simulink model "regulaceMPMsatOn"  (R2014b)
settings: Solver=ode45  StartTime=0.0  StopTime=50  RelTol=1e-3
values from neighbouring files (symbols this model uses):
  par = [0.2728 0.1079 0.3077 0.0546 0.1370 0.0320 0.1151 0.0357]    [regulaceMPM.m]    (also in SITOrizeniP.m = [-0.0536 0.05 0.13 0.006 -0.0545 0.1 0.16 0.1746 -0.058     ; SITOrizeniPD.m = [-0.0536 0.05 0.13 0.006 -0.0545 0.1 0.16 0.1746 -0.058     ; regulace1DoF.m; regulace2DoF.m)
undefined symbols (not defined in the file or in its folder): D, magnitude, N, P
libraries: simulink x8

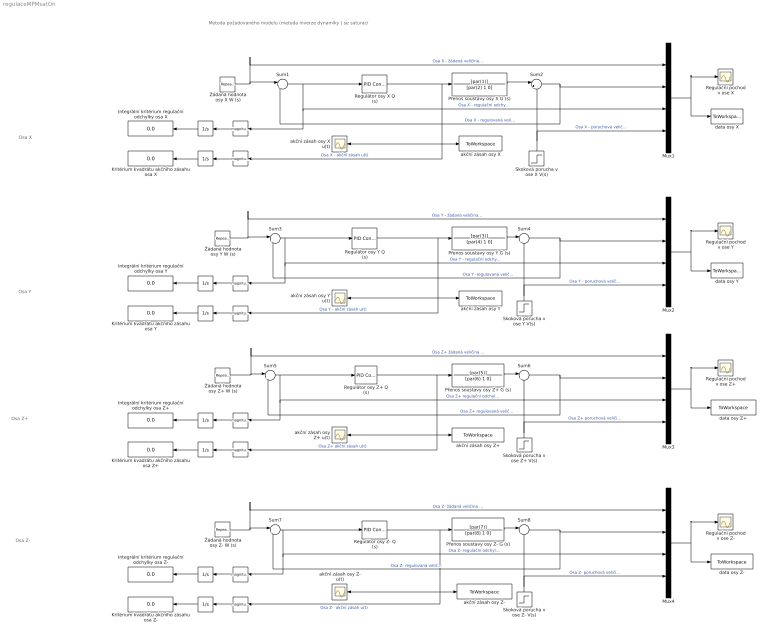
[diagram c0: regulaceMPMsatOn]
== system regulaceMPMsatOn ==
  note: Osa X
  note: Metoda požadovaného modelu (metoda inverze dynamiky ) se saturací
  note: Osa Y
  note: Osa Z+
  note: Osa Z-
  " " : Math  Operator=magnitude^2
  "  " : Integrator
  "   " : Integrator
  "     " : Integrator
  "      " : Math  Operator=magnitude^2
  "       " : Math  Operator=magnitude^2
  "        " : Integrator
  "          " : Integrator
  "           " : Math  Operator=magnitude^2
  "             " : Math  Operator=magnitude^2
  "              " : Integrator
  "                 " : Math  Operator=magnitude^2
  "                            " : Integrator
  "                               " : Math  Operator=magnitude^2
  "                                     " : Math  Operator=magnitude^2
  "                                       " : Integrator
  Integrální kritérium regulační odchylky osa X : Display
  Integrální kritérium regulační odchylky osa Y : Display
  Integrální kritérium regulační odchylky osa Z+ : Display
  Integrální kritérium regulační odchylky osa Z- : Display
  Kritérium kvadrátu akčního zásahu osa X : Display
  Kritérium kvadrátu akčního zásahu osa Y : Display
  Kritérium kvadrátu akčního zásahu osa Z+ : Display
  Kritérium kvadrátu akčního zásahu osa Z- : Display
  Mux{1..4} (4 alike) : Mux
  Přenos soustavy osy X G (s) : TransferFcn  Numerator=[par(1)]  Denominator=[par(2) 1 0]
  Přenos soustavy osy Y G (s) : TransferFcn  Numerator=[par(3)]  Denominator=[par(4) 1 0]
  Přenos soustavy osy Z+ G (s) : TransferFcn  Numerator=[par(5)]  Denominator=[par(6) 1 0]
  Přenos soustavy osy Z- G (s) : TransferFcn  Numerator=[par(7)]  Denominator=[par(8) 1 0]
  Regulační pochod v ose X : Scope
  Regulační pochod v ose Y : Scope
  Regulační pochod v ose Z+ : Scope
  Regulační pochod v ose Z- : Scope
  Regulátor osy X Q (s) : simulink/Continuous/PID Controller  Controller=PID  TimeDomain=Continuous-time  SampleTime=-1  IntegratorMethod=Forward Euler  FilterMethod=Forward Euler  Form=Parallel  P=P(1)  I=0  D=D(1)  N=N(1)  InitialConditionSource=internal  InitialConditionForIntegrator=0  InitialConditionForFilter=0  ExternalReset=none  LimitOutput=on  UpperSaturationLimit=1  LowerSaturationLimit=-1  LinearizeAsGain=on  AntiWindupMode=clamping  Kb=1  TrackingMode=off  Kt=1  PParamMin=[]  PParamMax=[]  IParamMin=[]  IParamMax=[]  DParamMin=[]  DParamMax=[]  NParamMin=[]  NParamMax=[]  KbParamMin=[]  KbParamMax=[]  KtParamMin=[]  KtParamMax=[]  POutMin=[]  POutMax=[]  IOutMin=[]  IOutMax=[]  DOutMin=[]  DOutMax=[]  NOutMin=[]  NOutMax=[]  KbOutMin=[]  KbOutMax=[]  KtOutMin=[]  KtOutMax=[]  IntegratorOutMin=[]  IntegratorOutMax=[]  FilterOutMin=[]  FilterOutMax=[]  SumOutMin=[]  SumOutMax=[]  SumI1OutMin=[]  SumI1OutMax=[]  SumI2OutMin=[]  SumI2OutMax=[]  SumI3OutMin=[]  SumI3OutMax=[]  SumDOutMin=[]  SumDOutMax=[]  SaturationOutMin=[]  SaturationOutMax=[]  IntegratorContinuousStateAttributes=''  IntegratorStateMustResolveToSignalObject=off  IntegratorRTWStateStorageClass=Auto  FilterContinuousStateAttributes=''  FilterStateMustResolveToSignalObject=off  FilterRTWStateStorageClass=Auto  DifferentiatorICPrevScaledInput=0  DifferentiatorOutMin=[]  DifferentiatorOutMax=[]  UseFilter=on
  Regulátor osy Y Q (s) : simulink/Continuous/PID Controller  Controller=PID  TimeDomain=Continuous-time  SampleTime=-1  IntegratorMethod=Forward Euler  FilterMethod=Forward Euler  Form=Parallel  P=P(2)  I=0  D=D(2)  N=N(2)  InitialConditionSource=internal  InitialConditionForIntegrator=0  InitialConditionForFilter=0  ExternalReset=none  LimitOutput=on  UpperSaturationLimit=1  LowerSaturationLimit=-1  LinearizeAsGain=on  AntiWindupMode=clamping  Kb=1  TrackingMode=off  Kt=1  PParamMin=[]  PParamMax=[]  IParamMin=[]  IParamMax=[]  DParamMin=[]  DParamMax=[]  NParamMin=[]  NParamMax=[]  KbParamMin=[]  KbParamMax=[]  KtParamMin=[]  KtParamMax=[]  POutMin=[]  POutMax=[]  IOutMin=[]  IOutMax=[]  DOutMin=[]  DOutMax=[]  NOutMin=[]  NOutMax=[]  KbOutMin=[]  KbOutMax=[]  KtOutMin=[]  KtOutMax=[]  IntegratorOutMin=[]  IntegratorOutMax=[]  FilterOutMin=[]  FilterOutMax=[]  SumOutMin=[]  SumOutMax=[]  SumI1OutMin=[]  SumI1OutMax=[]  SumI2OutMin=[]  SumI2OutMax=[]  SumI3OutMin=[]  SumI3OutMax=[]  SumDOutMin=[]  SumDOutMax=[]  SaturationOutMin=[]  SaturationOutMax=[]  IntegratorContinuousStateAttributes=''  IntegratorStateMustResolveToSignalObject=off  IntegratorRTWStateStorageClass=Auto  FilterContinuousStateAttributes=''  FilterStateMustResolveToSignalObject=off  FilterRTWStateStorageClass=Auto  DifferentiatorICPrevScaledInput=0  DifferentiatorOutMin=[]  DifferentiatorOutMax=[]  UseFilter=on
  Regulátor osy Z+ Q (s) : simulink/Continuous/PID Controller  Controller=PID  TimeDomain=Continuous-time  SampleTime=-1  IntegratorMethod=Forward Euler  FilterMethod=Forward Euler  Form=Parallel  P=P(3)  I=0  D=D(3)  N=N(3)  InitialConditionSource=internal  InitialConditionForIntegrator=0  InitialConditionForFilter=0  ExternalReset=none  LimitOutput=on  UpperSaturationLimit=1  LowerSaturationLimit=-1  LinearizeAsGain=on  AntiWindupMode=clamping  Kb=1  TrackingMode=off  Kt=1  PParamMin=[]  PParamMax=[]  IParamMin=[]  IParamMax=[]  DParamMin=[]  DParamMax=[]  NParamMin=[]  NParamMax=[]  KbParamMin=[]  KbParamMax=[]  KtParamMin=[]  KtParamMax=[]  POutMin=[]  POutMax=[]  IOutMin=[]  IOutMax=[]  DOutMin=[]  DOutMax=[]  NOutMin=[]  NOutMax=[]  KbOutMin=[]  KbOutMax=[]  KtOutMin=[]  KtOutMax=[]  IntegratorOutMin=[]  IntegratorOutMax=[]  FilterOutMin=[]  FilterOutMax=[]  SumOutMin=[]  SumOutMax=[]  SumI1OutMin=[]  SumI1OutMax=[]  SumI2OutMin=[]  SumI2OutMax=[]  SumI3OutMin=[]  SumI3OutMax=[]  SumDOutMin=[]  SumDOutMax=[]  SaturationOutMin=[]  SaturationOutMax=[]  IntegratorContinuousStateAttributes=''  IntegratorStateMustResolveToSignalObject=off  IntegratorRTWStateStorageClass=Auto  FilterContinuousStateAttributes=''  FilterStateMustResolveToSignalObject=off  FilterRTWStateStorageClass=Auto  DifferentiatorICPrevScaledInput=0  DifferentiatorOutMin=[]  DifferentiatorOutMax=[]  UseFilter=on
  Regulátor osy Z- Q (s) : simulink/Continuous/PID Controller  Controller=PID  TimeDomain=Continuous-time  SampleTime=-1  IntegratorMethod=Forward Euler  FilterMethod=Forward Euler  Form=Parallel  P=P(4)  I=0  D=D(4)  N=N(4)  InitialConditionSource=internal  InitialConditionForIntegrator=0  InitialConditionForFilter=0  ExternalReset=none  LimitOutput=on  UpperSaturationLimit=1  LowerSaturationLimit=-1  LinearizeAsGain=on  AntiWindupMode=clamping  Kb=1  TrackingMode=off  Kt=1  PParamMin=[]  PParamMax=[]  IParamMin=[]  IParamMax=[]  DParamMin=[]  DParamMax=[]  NParamMin=[]  NParamMax=[]  KbParamMin=[]  KbParamMax=[]  KtParamMin=[]  KtParamMax=[]  POutMin=[]  POutMax=[]  IOutMin=[]  IOutMax=[]  DOutMin=[]  DOutMax=[]  NOutMin=[]  NOutMax=[]  KbOutMin=[]  KbOutMax=[]  KtOutMin=[]  KtOutMax=[]  IntegratorOutMin=[]  IntegratorOutMax=[]  FilterOutMin=[]  FilterOutMax=[]  SumOutMin=[]  SumOutMax=[]  SumI1OutMin=[]  SumI1OutMax=[]  SumI2OutMin=[]  SumI2OutMax=[]  SumI3OutMin=[]  SumI3OutMax=[]  SumDOutMin=[]  SumDOutMax=[]  SaturationOutMin=[]  SaturationOutMax=[]  IntegratorContinuousStateAttributes=''  IntegratorStateMustResolveToSignalObject=off  IntegratorRTWStateStorageClass=Auto  FilterContinuousStateAttributes=''  FilterStateMustResolveToSignalObject=off  FilterRTWStateStorageClass=Auto  DifferentiatorICPrevScaledInput=0  DifferentiatorOutMin=[]  DifferentiatorOutMax=[]  UseFilter=on
  Skoková porucha v ose X V(s) : Step  Time=15  After=0.1  SampleTime=0
  Skoková porucha v ose Y V(s) : Step  Time=15  After=0.1  SampleTime=0
  Skoková porucha v ose Z+ V(s) : Step  Time=15  After=0.1  SampleTime=0
  Skoková porucha v ose Z- V(s) : Step  Time=15  After=0.1  SampleTime=0
  Sum{1,3,5,7} (4 alike) : Sum  Inputs=|+-
  Sum{2,4,6,8} (4 alike) : Sum  Inputs=|++
  akční zásah osy X : ToWorkspace  VariableName=akcniZasahXsat  SaveFormat=Timeseries  SampleTime=-1
  akční zásah osy X u(t) : Scope
  akční zásah osy Y : ToWorkspace  VariableName=akcniZasahYsat  SaveFormat=Timeseries  SampleTime=-1
  akční zásah osy Y u(t) : Scope
  akční zásah osy Z+ : ToWorkspace  VariableName=akcniZasahZplusSat  SaveFormat=Timeseries  SampleTime=-1
  akční zásah osy Z+ u(t) : Scope
  akční zásah osy Z- : ToWorkspace  VariableName=akcniZasahZminusSat  SaveFormat=Timeseries  SampleTime=-1
  akční zásah osy Z- u(t) : Scope
  data osy X : ToWorkspace  VariableName=dataXsat  SaveFormat=Timeseries  SampleTime=-1
  data osy Y : ToWorkspace  VariableName=dataYsat  SaveFormat=Timeseries  SampleTime=-1
  data osy Z+ : ToWorkspace  VariableName=dataZplusSat  SaveFormat=Timeseries  SampleTime=-1
  data osy Z- : ToWorkspace  VariableName=dataZminusSat  SaveFormat=Timeseries  SampleTime=-1
  Žádaná hodnota osy X W (s) : simulink/Sources/Repeating Sequence  rep_seq_t=[0 9.99 10 19.99 20 29.99 30 39.99 40 50]  rep_seq_y=[0 0 0.4 0.4 0.2 0.2 0.6 0.6 0 0]
  Žádaná hodnota osy Y W (s) : simulink/Sources/Repeating Sequence  rep_seq_t=[0 9.99 10 19.99 20 29.99 30 39.99 40 50]  rep_seq_y=[0 0 0.4 0.4 0.2 0.2 0.6 0.6 0 0]
  Žádaná hodnota osy Z+ W (s) : simulink/Sources/Repeating Sequence  rep_seq_t=[0 9.99 10 19.99 20 29.99 30 39.99 40 50]  rep_seq_y=[0 0 0.4 0.4 0.2 0.2 0.6 0.6 0 0]
  Žádaná hodnota osy Z- W (s) : simulink/Sources/Repeating Sequence  rep_seq_t=[0 9.99 10 19.99 20 29.99 30 39.99 40 50]  rep_seq_y=[0 0 0.4 0.4 0.2 0.2 0.6 0.6 0 0]
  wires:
  Žádaná hodnota osy X W (s)/1 -> Sum1/1, Mux1/1  "Osa X - žádaná veličina  w(t)"
  Sum1/1 -> Regulátor osy X Q (s)/1, "      "/1, Mux1/3  "Osa X - regulační odchylka e(t)"
  Přenos soustavy osy X G (s)/1 -> Sum2/1
  Sum2/1 -> Sum1/2, Mux1/2  "Osa X - regulovaná veličina y(t)"
  Skoková porucha v ose X V(s)/1 -> Sum2/2, Mux1/4  "Osa X - poruchová veličina v(t)"
  Mux1/1 -> data osy X/1, Regulační pochod v ose X/1
  "      "/1 -> "  "/1
  "  "/1 -> Integrální kritérium regulační odchylky osa X/1
  "     "/1 -> Kritérium kvadrátu akčního zásahu osa X/1
  " "/1 -> "     "/1
  Žádaná hodnota osy Y W (s)/1 -> Sum3/1, Mux2/1  "Osa Y - žádaná veličina w(t)"
  Sum3/1 -> Regulátor osy Y Q (s)/1, Mux2/3, "                                     "/1  "Osa Y - regulační odchylka e(t)"
  Přenos soustavy osy Y G (s)/1 -> Sum4/1
  Sum4/1 -> Sum3/2, Mux2/2  "Osa Y -regulovaná veličina y(t)"
  Skoková porucha v ose Y V(s)/1 -> Mux2/4, Sum4/2  "Osa Y - poruchová veličina v(t)"
  Mux2/1 -> data osy Y/1, Regulační pochod v ose Y/1
  "                                     "/1 -> "                            "/1
  "                            "/1 -> Integrální kritérium regulační odchylky osa Y/1
  "                                       "/1 -> Kritérium kvadrátu akčního zásahu osa Y/1
  "                               "/1 -> "                                       "/1
  Žádaná hodnota osy Z+ W (s)/1 -> Sum5/1, Mux3/1  "Osa Z+ žádaná veličina  w(t)"
  Sum5/1 -> Regulátor osy Z+ Q (s)/1, "                 "/1, Mux3/3  "Osa Z+ regulační odchylka e(t)"
  Přenos soustavy osy Z+ G (s)/1 -> Sum6/1
  Sum6/1 -> Sum5/2, Mux3/2  "Osa Z+ regulovaná veličina y(t)"
  Skoková porucha v ose Z+ V(s)/1 -> Sum6/2, Mux3/4  "Osa Z+ poruchová veličina v(t)"
  Mux3/1 -> data osy Z+/1, Regulační pochod v ose Z+/1
  "                 "/1 -> "          "/1
  "          "/1 -> Integrální kritérium regulační odchylky osa Z+/1
  "              "/1 -> Kritérium kvadrátu akčního zásahu osa Z+/1
  "           "/1 -> "              "/1
  Žádaná hodnota osy Z- W (s)/1 -> Sum7/1, Mux4/1  "Osa Z- žádaná veličina w(t)"
  Sum7/1 -> Regulátor osy Z- Q (s)/1, Mux4/3, "             "/1  "Osa Z- regulační odchylka e(t)"
  Přenos soustavy osy Z- G (s)/1 -> Sum8/1
  Sum8/1 -> Sum7/2, Mux4/2  "Osa Z- regulovaná veličina y(t)"
  Mux4/1 -> data osy Z-/1, Regulační pochod v ose Z-/1
  "             "/1 -> "   "/1
  "   "/1 -> Integrální kritérium regulační odchylky osa Z-/1
  "        "/1 -> Kritérium kvadrátu akčního zásahu osa Z-/1
  "       "/1 -> "        "/1
  Regulátor osy X Q (s)/1 -> akční zásah osy X/1, akční zásah osy X u(t)/1, " "/1, Přenos soustavy osy X G (s)/1  "Osa X - akční zásah u(t)"
  Regulátor osy Y Q (s)/1 -> akční zásah osy Y/1, akční zásah osy Y u(t)/1, "                               "/1, Přenos soustavy osy Y G (s)/1  "Osa Y - akční zásah u(t)"
  Regulátor osy Z+ Q (s)/1 -> akční zásah osy Z+/1, akční zásah osy Z+ u(t)/1, "           "/1, Přenos soustavy osy Z+ G (s)/1  "Osa Z+ akční zásah u(t)"
  Regulátor osy Z- Q (s)/1 -> akční zásah osy Z- u(t)/1, akční zásah osy Z-/1, "       "/1, Přenos soustavy osy Z- G (s)/1  "Osa Z-  akční zásah u(t)"
  Skoková porucha v ose Z- V(s)/1 -> Mux4/4, Sum8/2  "Osa Z- poruchová veličina v(t)"
